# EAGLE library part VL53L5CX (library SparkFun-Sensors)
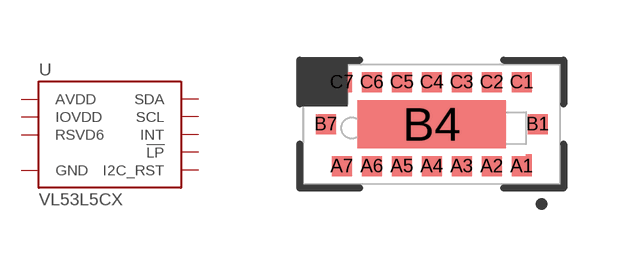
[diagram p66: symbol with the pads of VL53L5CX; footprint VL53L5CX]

Designator prefix U

## VL53L5CX (PROD_ID: IC-16254)  [VL53L5CX]
A1  I2C_RST
A2  GND
A3  INT
A4  IOVDD
A5  !LP
A6  GND
A7  GND
B1  AVDD
B4  GND
B7  AVDD
C1  GND
C2  RSVD6
C3  SDA
C4  SCL
C6  GND
C7  GND

## Footprint VL53L5CX (pad centres in mm)
smd 0.5 x 0.5: A1 2.25,-1.05; A2 1.5,-1.05; A3 0.75,-1.05; A4 0,-1.05; A5 -0.75,-1.05; A6 -1.5,-1.05; A7 -2.25,-1.05; B1 2.65,0; B7 -2.65,0; C1 2.25,1.05; C2 1.5,1.05; C3 0.75,1.05; C4 0,1.05; C5 -0.75,1.05; C6 -1.5,1.05; C7 -2.25,1.05
smd 3.7 x 1.2: B4 0,0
